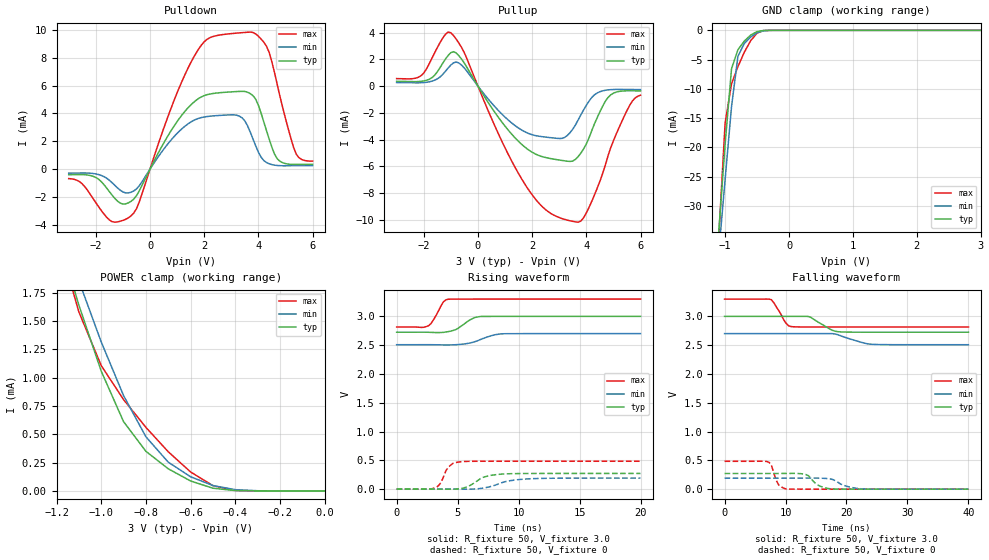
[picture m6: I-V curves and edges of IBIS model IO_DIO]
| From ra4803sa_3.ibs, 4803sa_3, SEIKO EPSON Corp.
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[Model]   IO_DIO
Model_type I/O
Enable Active-High
Polarity Non-Inverting
Vinh=2.4
Vinl=0.6
Vmeas=1.50
C_comp   5p   4p   6p
[Temperature Range] 25   85   -40
[Voltage Range]   3.0   2.7   3.3
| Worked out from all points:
|   slope of the pulldown table from 0 to 0.45 V, typ, clamps not added: 268 ohm
|   slope of the pullup table from 0 to 0.45 V, typ, clamps not added: 311 ohm
|   GND clamp passes 1 mA (typ) near -0.62 V on its own axis
|   POWER clamp passes 1 mA (typ) near -0.99 V on its own axis
|   falling waveform, R_fixture 50, V_fixture 3.0: 20-80 % time 2.59ns typ, 3.46ns min, 1.61ns max; typ from 3 V to 2.72 V
|   falling waveform, R_fixture 50, V_fixture 0: 20-80 % time 1.74ns typ, 2.43ns min, 993ps max; typ from 0.272 V to 0 V
|   rising waveform, R_fixture 50, V_fixture 3.0: 20-80 % time 1.15ns typ, 1.55ns min, 763ps max; typ from 2.72 V to 3 V
|   rising waveform, R_fixture 50, V_fixture 0: 20-80 % time 1.36ns typ, 1.95ns min, 704ps max; typ from 0 V to 0.272 V
[Pullup]
-3V       358.5uA    266uA      560.5uA
-2.1V     355.6uA    250.6uA    776.4uA
-1V       2.502mA    1.574mA    3.995mA
-600mV    2.01mA     1.562mA    2.877mA
800mV     -2.466mA   -1.922mA   -3.767mA
1.8V      -4.673mA   -3.487mA   -7.55mA
3.1V      -5.565mA   -3.917mA   -9.914mA
3.7V      -5.274mA   -2.526mA   -10.19mA
4.2V      -3.339mA   -856.1uA   -8.631mA
4.8V      -856uA     -284.2uA   -5.227mA
5.6V      -352.1uA   -256.3uA   -1.441mA
6V        -359.4uA   -261.7uA   -678.8uA
[Pulldown]
-3V       -406.7uA   -291.8uA   -681.1uA
-2V       -601.3uA   -346.1uA   -2.408mA
-1.4V     -1.867mA   -974.9uA   -3.772mA
-700mV    -2.315mA   -1.662mA   -3.357mA
900mV     3.128mA    2.362mA    4.993mA
1.8V      5.08mA     3.65mA     8.644mA
3.6V      5.522mA    3.109mA    9.832mA
3.9V      5.025mA    1.678mA    9.709mA
4.3V      2.754mA    473.4uA    8.824mA
4.7V      732.6uA    259.2uA    6.038mA
5.4V      334.3uA    244.3uA    1.067mA
6V        344.9uA    252.2uA    575.7uA
[GND Clamp]
-3V       -337.8mA   -292.1mA   -428.7mA
-1.1V     -34.38mA   -38.01mA   -35.33mA
-1V       -19.42mA   -25.43mA   -15.8mA
-900mV    -6.562mA   -13.04mA   -9.129mA
-800mV    -3.309mA   -4.443mA   -6.201mA
-700mV    -1.841mA   -2.238mA   -3.742mA
-600mV    -807.8uA   -1.13mA    -1.764mA
-500mV    -207.4uA   -422.3uA   -476.4uA
-400mV    -22.76uA   -87.36uA   -42.64uA
-300mV    -1.222uA   -9.219uA   -1.241uA
3V        69.12pA    1.595uA    45.25pA
[POWER Clamp]
-3V       16.37mA    14.49mA    19.53mA
-1.2V     2.299mA    2.435mA    2.272mA
-1.1V     1.642mA    1.856mA    1.581mA
-1V       1.058mA    1.316mA    1.108mA
-900mV    611.8uA    841.8uA    806.6uA
-800mV    349.6uA    477.9uA    561.1uA
-700mV    195.4uA    253.6uA    345.8uA
-600mV    87.51uA    124.8uA    167uA
-500mV    23.8uA     47.35uA    46.11uA
-400mV    3.184uA    11.02uA    4.195uA
-300mV    282.7nA    1.595uA    173.3nA
0V        69.01pA    1.404nA    54.11pA
[Falling Waveform]
R_fixture=50
V_fixture=3.0
V_fixture_min=2.7
V_fixture_max=3.3
0s        3V         2.7V       3.3V
7.677ns   3V         2.7V       3.29V
10.1ns    3V         2.7V       2.878V
10.91ns   3V         2.7V       2.823V
13.74ns   2.998V     2.7V       2.815V
17.37ns   2.774V     2.701V     2.815V
18.59ns   2.734V     2.681V     2.815V
22.63ns   2.725V     2.544V     2.815V
24.24ns   2.724V     2.515V     2.815V
40ns      2.724V     2.508V     2.815V
[Falling Waveform]
R_fixture=50
V_fixture=0
V_fixture_min=0
V_fixture_max=0
0s        272.1mV    191.1mV    483.8mV
7.273ns   272.1mV    191.1mV    467.1mV
7.677ns   272.1mV    191.1mV    419.2mV
8.889ns   272.4mV    191.1mV    72.17mV
10.1ns    272.8mV    191.2mV    3.752mV
13.33ns   253.3mV    191.8mV    51.32uV
15.35ns   68.66mV    191.6mV    19.53uV
17.78ns   1.885mV    166.3mV    -13.77uV
22.63ns   9.422uV    4.666mV    -5.093uV
40ns      -4.67uV    25.67uV    7.491uV
[Rising Waveform]
R_fixture=50
V_fixture=3.0
V_fixture_min=2.7
V_fixture_max=3.3
0s        2.724V     2.508V     2.815V
2.626ns   2.723V     2.508V     2.839V
3.03ns    2.72V      2.507V     2.945V
3.838ns   2.722V     2.503V     3.253V
4.242ns   2.735V     2.503V     3.298V
4.848ns   2.77V      2.507V     3.299V
5.859ns   2.918V     2.531V     3.3V
6.869ns   2.997V     2.597V     3.3V
8.687ns   3V         2.697V     3.3V
20ns      3V         2.7V       3.3V
[Rising Waveform]
R_fixture=50
V_fixture=0
V_fixture_min=0
V_fixture_max=0
0s        0V         0V         0V
3.232ns   60uV       64.13uV    27.95mV
3.636ns   -50.56uV   66.59uV    114.8mV
4.242ns   -536.9uV   1.042uV    381.2mV
4.646ns   -241.4uV   -93.67uV   451.2mV
5.253ns   9.834mV    -392.6uV   474.5mV
7.071ns   202.3mV    17.07mV    483.7mV
8.283ns   255.2mV    84.71mV    483.8mV
11.11ns   271.6mV    181.1mV    483.8mV
20ns      272.1mV    191.1mV    483.8mV
[Ramp]
R_load=50
dV/dt_r   1.632E-1/1.351E-9   1.147E-1/1.940E-9   2.903E-1/6.904E-10
dV/dt_f   1.640E-1/2.550E-9   4.377E-2/1.133E-9   2.909E-1/1.597E-9
|[End   IO_DIO
